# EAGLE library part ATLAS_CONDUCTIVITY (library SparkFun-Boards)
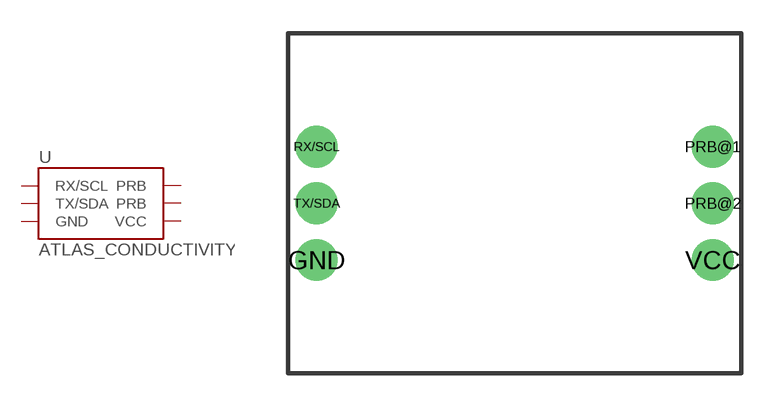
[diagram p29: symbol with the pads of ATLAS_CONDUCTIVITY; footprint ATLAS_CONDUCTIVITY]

Designator prefix U

## ATLAS_CONDUCTIVITY  [ATLAS_CONDUCTIVITY]
GND  GND  pwr
PRB@1  PRB
PRB@2  PRB
RX/SCL  RX/SCL
TX/SDA  TX/SDA
VCC  VCC  pwr

## Footprint ATLAS_CONDUCTIVITY (pad centres in mm)
drill 1.118 pad 1.88: GND 1.27,5.08; PRB@1 19.05,10.16; PRB@2 19.05,7.62; RX/SCL 1.27,10.16; TX/SDA 1.27,7.62; VCC 19.05,5.08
